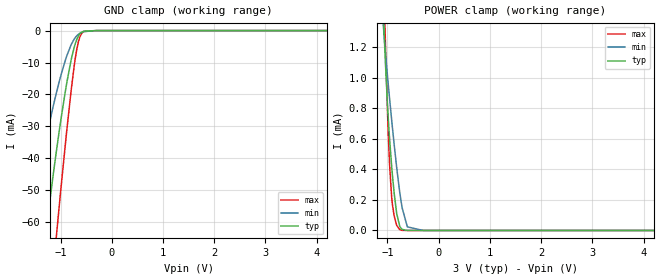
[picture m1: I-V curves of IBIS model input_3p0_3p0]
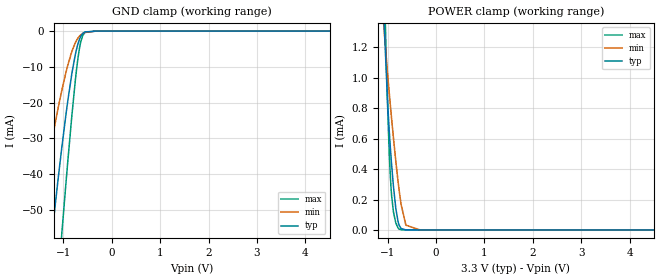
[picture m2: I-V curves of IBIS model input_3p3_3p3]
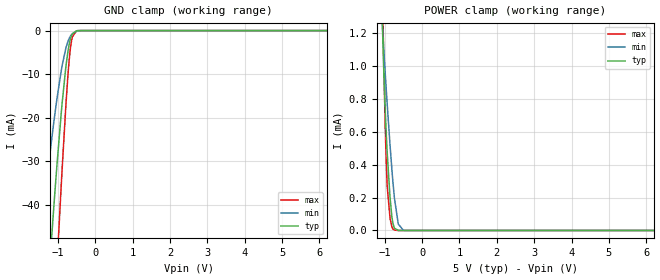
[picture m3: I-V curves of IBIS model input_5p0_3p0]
|Texas Instruments Incorporated
| ADS124S0x Low-Power, Low-Noise, Highly-Integrated, 6- and 12-Channel,4-kSPS,
| 24-Bit, Delta-Sigma ADC with PGA and Voltage Reference
| Marketing part#   Digital Voltage Range   Package-type   #pins
| ADS124S08IPBS   2.7V-5.25V   TQFP   32
| ADS124S08IPBSR   2.7V-5.25V   TQFP   32
| ADS124S08IRHBT   2.7V-5.25V   VQFN   32
| ADS124S08IRHBR   2.7V-5.25V   VQFN   32
[IBIS Ver]   4.1
[File name]   ads124s08.ibs
[File Rev]   2.0
[Date]   10/17/2016
[Source]
| Texas Instruments Incorporated.
| Analog-eLab Design Center, HPA
| 12500 TI Blvd
| Dallas, TX -75243
[Notes]   Revision History:
| Rev 2.0: 10/17/2016
| - input_*,csn_*,output_* Voltage range changed.
| Rev 1.0: 9/17/2016
| - Initial version of the model
| - Model generated from simulations in SPECTRE
| - Model matched to SPICE simulation
| - C_comp although listed in numerical order of value are
|   obtained from varying PVT conditions. For PVT conditions for
|   each specific value refer the buffer description under
|   respective [Model]. IBIS model user is responsible for using
|   appropriate C_comp to simulate for Signal Integrity.
|*Exception:   *
|* Pullup and Pulldown currents of output buffer are not passing through  *
|* zero because of drive switchs (MP13,MP12,MP14,MP15,MP10,MP11,MP0,MP2,  *
|* MP1,MP3,MP16,MP17 and MN12,MN11,MN13,MN14,MN5,MN6,MN4,MN3 respectively)*
|* arrangement   *
|[Disclaimer]
| This model is designed as an aid for customers of Texas Instruments.
| TI and its licensors and suppliers make no warranties, either expressed
| or implied, with respect to this  model, including the warranties of
| merchantability or fitness for a particular purpose. The model is
| provided solely on an "as is" basis. The entire risk as to its quality
| and performance is with the customer.
[Copyright]
(C) Copyright 2016 Texas Instruments Incorporated.All rights reserved.
|   ADS124S08PBS
[Component]   ADS124S08PBS
[Manufacturer]   TI
[Package]   |32 TQFP  -  PBS package
|   typ   min   max
R_pkg   0.1   0.08   0.12
L_pkg   1.0nH   0.8nH   1.2nH
C_pkg   0.2pF   0.16pF   0.24pF
[Pin]  signal_name   model_name   R_pin   L_pin   C_pin
1   AINCOM   NC   NA   NA   NA
2   AIN5   NC   NA   NA   NA
3   AIN4   NC   NA   NA   NA
4   AIN3   NC   NA   NA   NA
5   AIN2   NC   NA   NA   NA
6   AIN1   NC   NA   NA   NA
7   AIN0   NC   NA   NA   NA
8   START/SYNC   INPUT   NA   NA   NA
9   CS   CSN   NA   NA   NA
10   DIN   INPUT   NA   NA   NA
11   SCLK   INPUT   NA   NA   NA
12   DOUT/_DRDY   OUTPUT   NA   NA   NA
13   _DRDY   OUTPUT   NA   NA   NA
14   DGND   GND   NA   NA   NA
15   IOVDD   POWER   NA   NA   NA
16   DVDD   POWER   NA   NA   NA
17   CLK   INPUT   NA   NA   NA
18   _RESET   INPUT   NA   NA   NA
19   GPIO3/AIN11   NC   NA   NA   NA
20   GPIO2/AIN10   NC   NA   NA   NA
21   GPIO1/AIN9   NC   NA   NA   NA
22   GPIO0/AIN8   NC   NA   NA   NA
23   REFOUT   NC   NA   NA   NA
24   REFCOM   NC   NA   NA   NA
25   NC   NC   NA   NA   NA
26   AVDD   POWER   NA   NA   NA
27   AVSS   GND   NA   NA   NA
28   AVSS-SW   GND   NA   NA   NA
29   REFN0   NC   NA   NA   NA
30   REFP0   NC   NA   NA   NA
31   REFN1/AIN7   NC   NA   NA   NA
32   REFP1/AIN6   NC   NA   NA   NA
33   ThermalPad   NC   NA   NA   NA
|   ADS124S08RHB
[Component]   ADS124S08RHB
[Manufacturer]   TI
[Package]   |32 VQFN  -  RHB package
|   typ   min   max
R_pkg   0.1   0.08   0.12
L_pkg   1.0nH   0.8nH   1.2nH
C_pkg   0.2pF   0.16pF   0.24pF
[Pin]  signal_name   model_name   R_pin   L_pin   C_pin
1   AINCOM   NC   NA   NA   NA
2   AIN5   NC   NA   NA   NA
3   AIN4   NC   NA   NA   NA
4   AIN3   NC   NA   NA   NA
5   AIN2   NC   NA   NA   NA
6   AIN1   NC   NA   NA   NA
7   AIN0   NC   NA   NA   NA
8   START/SYNC   INPUT   NA   NA   NA
9   CS   CSN   NA   NA   NA
10   DIN   INPUT   NA   NA   NA
11   SCLK   INPUT   NA   NA   NA
12   DOUT/_DRDY   OUTPUT   NA   NA   NA
13   _DRDY   OUTPUT   NA   NA   NA
14   DGND   GND   NA   NA   NA
15   IOVDD   POWER   NA   NA   NA
16   DVDD   POWER   NA   NA   NA
17   CLK   INPUT   NA   NA   NA
18   _RESET   INPUT   NA   NA   NA
19   GPIO3/AIN11   NC   NA   NA   NA
20   GPIO2/AIN10   NC   NA   NA   NA
21   GPIO1/AIN9   NC   NA   NA   NA
22   GPIO0/AIN8   NC   NA   NA   NA
23   REFOUT   NC   NA   NA   NA
24   REFCOM   NC   NA   NA   NA
25   NC   NC   NA   NA   NA
26   AVDD   POWER   NA   NA   NA
27   AVSS   GND   NA   NA   NA
28   AVSS-SW   GND   NA   NA   NA
29   REFN0   NC   NA   NA   NA
30   REFP0   NC   NA   NA   NA
31   REFN1/AIN7   NC   NA   NA   NA
32   REFP1/AIN6   NC   NA   NA   NA
33   ThermalPad   NC   NA   NA   NA
|   Model Selectors
[Model Selector] INPUT
input_3p0_3p0   3.0V  digital Input
input_3p3_3p3   3.3V  digital Input
input_5p0_3p0   5.0V  digital Input,  internal 3.0V DVDD
input_5p0_3p3   5.0V  digital Input,  internal 3.3V DVDD
[Model Selector] CSN
csn_3p0_3p0   3.0V  digital Input
csn_3p3_3p3   3.3V  digital Input
csn_5p0_3p0   5.0V  digital Input,  internal 3.0V DVDD
csn_5p0_3p3   5.0V  digital Input,  internal 3.3V DVDD
[Model Selector] OUTPUT
output_3p0_3p0   3.0V  digital Output
output_3p3_3p3   3.3V  digital Output
output_5p0_3p0   5.0V  digital Output, internal 3.0V DVDD
output_5p0_3p3   5.0V  digital Output, internal 3.3V DVDD
| Models and submodels in the file (12): input_3p0_3p0 (Input), input_3p3_3p3 (Input), input_5p0_3p0 (Input), input_5p0_3p3 (Input), csn_3p0_3p0 (Input), csn_3p3_3p3 (Input), csn_5p0_3p0 (Input), csn_5p0_3p3 (Input), output_3p0_3p0 (Output), output_3p3_3p3 (Output), output_5p0_3p0 (Output), output_5p0_3p3 (Output)
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|   input_3p0_3p0 Model
[Model]   input_3p0_3p0
Model_type   Input
Vinl = 0.9
Vinh = 2.1
|   typ   min   max
|   (nom PVT)   (fast PVT)   (slow PVT)
C_comp   2.012e-12   1.852e-12   2.193e-12
[Model spec]
|subparameter
Vinl   0.90   0.81   0.99
Vinh   2.10   1.89   2.31
| Where nom  PVT is Nominal Process, 3V, 27C
|   Fast PVT is Strong Process,  3.3V, -50C
|   Slow PVT is Weak Process,   2.7V, 125C
[Voltage Range]   3   2.7   3.3
|Junction Temperature
[Temperature Range]   27   125   -50
[Power Clamp Reference]   3   2.7   3.3
[GND Clamp Reference]   0   0   0
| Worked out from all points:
|   GND clamp passes 1 mA (typ) near -0.62 V on its own axis
|   POWER clamp passes 1 mA (typ) near -1.02 V on its own axis
[GND Clamp]
|   Voltage   I(typ)   I(min)   I(max)
-3V       -319mA     -211mA     -412.6mA
-1.627V   -110.2mA   -63.4mA    -162.1mA
-1.294V   -64.19mA   -34.85mA   -101.7mA
-1.245V   -57.9mA    -31.12mA   -93.07mA
-1.076V   -37.25mA   -19.22mA   -63.58mA
-879mV    -16.48mA   -7.979mA   -31.47mA
-736.2mV  -5.413mA   -2.751mA   -11.46mA
-683.4mV  -2.806mA   -1.644mA   -5.954mA
-648mV    -1.608mA   -1.128mA   -3.314mA
-582mV    -428.1uA   -525.1uA   -758.2uA
-300mV    -151.4nA   -2.235uA   -33.79nA
6V        0A         0A         0A
[POWER Clamp]
|   Voltage   I(typ)   I(min)   I(max)
-3V       26.48mA    20.48mA    33.5mA
-1.107V   1.693mA    1.467mA    2.138mA
-1.064V   1.301mA    1.272mA    1.554mA
-1.044V   1.137mA    1.189mA    1.298mA
-980.4mV  719uA      946.5uA    611.5uA
-957mV    598.7uA    862.9uA    428.5uA
-917.7mV  425.1uA    727.2uA    222.8uA
-819mV    112.3uA    413uA      33.86uA
-756mV    25.23uA    242.6uA    4.514uA
-610.5mV  291.5nA    23.53uA    29.55nA
-300mV    0A         0A         0A
6V        0A         0A         0A
|   input_3p3_3p3 Model
[Model]   input_3p3_3p3
Model_type   Input
Vinl = 0.99
Vinh = 2.31
|   typ   min   max
|   (nom PVT)   (fast PVT)   (slow PVT)
C_comp   2.012e-12   1.852e-12   2.130e-12
[Model spec]
|subparameter
Vinl   0.99   0.90   1.08
Vinh   2.31   2.10   2.52
| Where nom  PVT is Nominal Process, 3.3V, 27C
|   Fast PVT is Strong Process,  3.6V, -50C
|   Slow PVT is Weak Process,   3V, 125C
[Voltage Range]   3.3   3   3.6
|Junction Temperature
[Temperature Range]   27   125   -50
[Power Clamp Reference]   3.3   3   3.6
[GND Clamp Reference]   0   0   0
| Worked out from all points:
|   GND clamp passes 1 mA (typ) near -0.62 V on its own axis
|   POWER clamp passes 1 mA (typ) near -1.02 V on its own axis
[GND Clamp]
|   Voltage   I(typ)   I(min)   I(max)
-3.3V     -365.9mA   -246.2mA   -467.2mA
-1.758V   -129.1mA   -75.74mA   -185.9mA
-1.495V   -91.39mA   -51.49mA   -138mA
-1.233V   -56.33mA   -30.2mA    -90.88mA
-1.04V    -33.04mA   -16.86mA   -57.33mA
-924mV    -20.77mA   -10.2mA    -38.44mA
-831mV    -12.21mA   -5.864mA   -24.24mA
-733.2mV  -5.222mA   -2.669mA   -11.07mA
-648mV    -1.6mA     -1.124mA   -3.296mA
-607.2mV  -735.4uA   -708uA     -1.402mA
-556.8mV  -236.3uA   -380.5uA   -378.8uA
6.6V      0A         0A         0A
[POWER Clamp]
|   Voltage   I(typ)   I(min)   I(max)
-3.3V     30.57mA    23.74mA    38.59mA
-1.082V   1.459mA    1.351mA    1.793mA
-1.057V   1.241mA    1.242mA    1.46mA
-1.01V    896.1uA    1.056mA    903.3uA
-967.2mV  647.9uA    898.1uA    500.5uA
-927.6mV  464.9uA    760uA      262uA
-879mV    280.1uA    598.2uA    115.3uA
-831mV    139.2uA    448uA      45.08uA
-765.6mV  32.61uA    265.8uA    6.266uA
-624mV    432.6nA    31.8uA     47.44nA
-330mV    0A         11.66nA    0A
6.6V      0A         0A         0A
|   input_5p0_3p0 Model
[Model]   input_5p0_3p0
Model_type   Input
Vinl = 1.5
Vinh = 3.5
|   typ   min   max
|   (nom PVT)   (fast PVT)   (slow PVT)
C_comp   1.956e-12   1.803e-12   2.130e-12
[Model spec]
|subparameter
Vinl   1.5   1.425   1.575
Vinh   3.5   3.325   3.675
| Where nom  PVT is Nominal Process, 5V, 27C
|   Fast PVT is Strong Process,  5.25V, -50C
|   Slow PVT is Weak Process,   4.75V, 125C
[Voltage Range]   5   4.75   5.25
|Junction Temperature
[Temperature Range]   27   125   -50
[Power Clamp Reference]   5   4.75   5.25
[GND Clamp Reference]   0   0   0
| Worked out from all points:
|   GND clamp passes 1 mA (typ) near -0.62 V on its own axis
|   POWER clamp passes 1 mA (typ) near -1.03 V on its own axis
[GND Clamp]
|   Voltage   I(typ)   I(min)   I(max)
-5V       -633.1mA   -452.9mA   -777.1mA
-1.446V   -84.35mA   -47.1mA    -128.8mA
-1.167V   -47.93mA   -25.3mA    -79.05mA
-1.115V   -41.58mA   -21.66mA   -69.92mA
-1.02V    -30.68mA   -15.55mA   -53.79mA
-905.5mV  -18.79mA   -9.165mA   -35.27mA
-777.2mV  -7.931mA   -3.86mA    -16.44mA
-695mV    -3.207mA   -1.813mA   -6.83mA
-658.5mV  -1.857mA   -1.237mA   -3.866mA
-610mV    -752.4uA   -716.9uA   -1.441mA
-497mV    -50.16uA   -160.2uA   -57.93uA
10V       0A         0A         0A
[POWER Clamp]
|   Voltage   I(typ)   I(min)   I(max)
-5V       53.84mA    42.33mA    67.58mA
-1.057V   1.228mA    1.235mA    1.44mA
-1.026V   988.5uA    1.109mA    1.056mA
-978.5mV  698.5uA    933uA      578.6uA
-945mV    533.9uA    814.6uA    341.7uA
-930mV    468.3uA    762.9uA    265.6uA
-855mV    199.2uA    517uA      72.4uA
-805.3mV  81.92uA    368.3uA    21.94uA
-737mV    13.7uA     194.9uA    2.163uA
-634.8mV  568.7nA    38.85uA    65.65nA
-478mV    0A         646.1nA    0A
10V       0A         0A         0A
